(* Logix 5000 AddOnInstructionDefinition export AMCI_3601_AOP_Absolute_Move; software revision 20.03 *)

ADD_ON_INSTRUCTION AMCI_3601_AOP_Absolute_Move   (* revision 0.0, vendor AMCI, ExecuteEnableInFalse *)
// Revision note:
// 3/2020: Version 0 is the initial release
VAR_INPUT
   Axis_Status_Bits : INT; {required}
   _0_normal_1_S_Curve_Acceleration : BOOL;
   _0_Triangular_1_Trapezoidal_S_Curve : BOOL;
   _0_Target_Move_1_Encoder_Move : BOOL;
   Target_Position : DINT; {required}
   Programmed_Speed : DINT; {required}
   Acceleration : INT; {required}
   Deceleration : INT; {required}
END_VAR
VAR_OUTPUT
   EN : BOOL; {access Read Only, visible}
   ER : BOOL; {access Read Only, visible}
END_VAR
VAR_IN_OUT
   AMCI_3601_output_data : AM:1769_3601:O:0; {required}
END_VAR
VAR
   Upper_Result_X_1000 : DINT;
   command_data_block : INT[10];
        [0]   // Command Bits MSW
        [1]   // Command Bits LSW
        [2]   // Upper Target Position
        [3]   // Lower Target Position
        [4]   // Upper Programmed Speed
        [5]   // Lower Programmed Speed
END_VAR

ROUTINE EnableInFalse   (* ladder *)
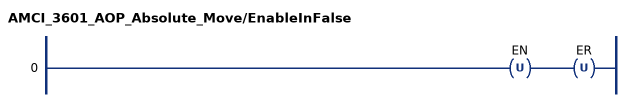
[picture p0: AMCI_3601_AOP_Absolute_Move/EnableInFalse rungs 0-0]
   0: OTU(EN)OTU(ER);
END_ROUTINE

ROUTINE Logic   (* ladder *)
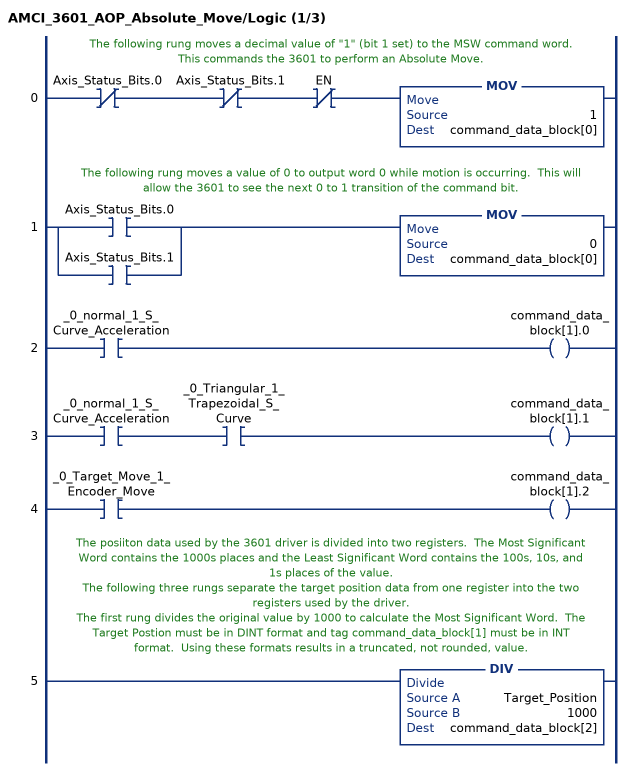
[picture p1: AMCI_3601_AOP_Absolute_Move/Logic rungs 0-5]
   // The following rung moves a decimal value of "1" (bit 1 set) to the MSW command word.  This commands the 3601 to perform an Absolute Move.
   0: XIO(Axis_Status_Bits.0)XIO(Axis_Status_Bits.1)XIO(EN)MOV(1,command_data_block[0]);
   // The following rung moves a value of 0 to output word 0 while motion is occurring.  This will allow the 3601 to see the next 0 to 1 transition of the command bit.
   1: [XIC(Axis_Status_Bits.0) ,XIC(Axis_Status_Bits.1) ]MOV(0,command_data_block[0]);
   2: XIC(_0_normal_1_S_Curve_Acceleration)OTE(command_data_block[1].0);
   3: XIC(_0_normal_1_S_Curve_Acceleration)XIC(_0_Triangular_1_Trapezoidal_S_Curve)OTE(command_data_block[1].1);
   4: XIC(_0_Target_Move_1_Encoder_Move)OTE(command_data_block[1].2);
   // The posiiton data used by the 3601 driver is divided into two registers.  The Most Significant Word contains the 1000s places and the Least Significant Word contains the 100s, 10s, and 1s places of the value.
   // The following three rungs separate the target position data from one register into the two registers used by the driver.
   // The first rung divides the original value by 1000 to calculate the Most Significant Word.  The Target Postion must be in DINT format and tag command_data_block[1] must be in INT format.  Using these formats results in a truncated, not rounded, value.
   5: DIV(Target_Position,1000,command_data_block[2]);
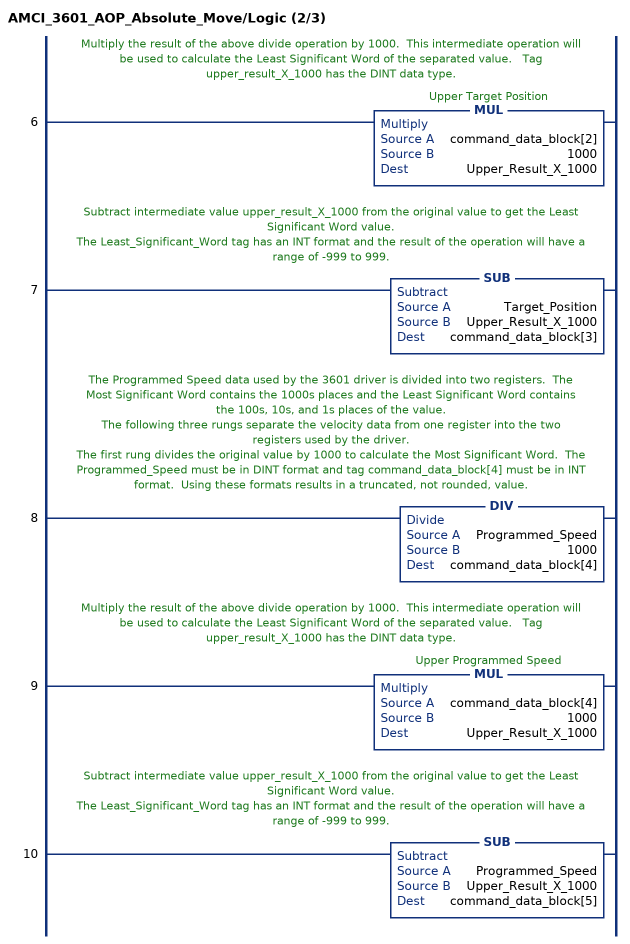
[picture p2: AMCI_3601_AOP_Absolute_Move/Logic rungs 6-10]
   // Multiply the result of the above divide operation by 1000.  This intermediate operation will be used to calculate the Least Significant Word of the separated value.   Tag upper_result_X_1000 has the DINT data type.
   6: MUL(command_data_block[2],1000,Upper_Result_X_1000);
   // Subtract intermediate value upper_result_X_1000 from the original value to get the Least Significant Word value.
   // The Least_Significant_Word tag has an INT format and the result of the operation will have a range of -999 to 999.
   7: SUB(Target_Position,Upper_Result_X_1000,command_data_block[3]);
   // The Programmed Speed data used by the 3601 driver is divided into two registers.  The Most Significant Word contains the 1000s places and the Least Significant Word contains the 100s, 10s, and 1s places of the value.
   // The following three rungs separate the velocity data from one register into the two registers used by the driver.
   // The first rung divides the original value by 1000 to calculate the Most Significant Word.  The Programmed_Speed must be in DINT format and tag command_data_block[4] must be in INT format.  Using these formats results in a truncated, not rounded, value.
   8: DIV(Programmed_Speed,1000,command_data_block[4]);
   // Multiply the result of the above divide operation by 1000.  This intermediate operation will be used to calculate the Least Significant Word of the separated value.   Tag upper_result_X_1000 has the DINT data type.
   9: MUL(command_data_block[4],1000,Upper_Result_X_1000);
   // Subtract intermediate value upper_result_X_1000 from the original value to get the Least Significant Word value.
   // The Least_Significant_Word tag has an INT format and the result of the operation will have a range of -999 to 999.
   10: SUB(Programmed_Speed,Upper_Result_X_1000,command_data_block[5]);
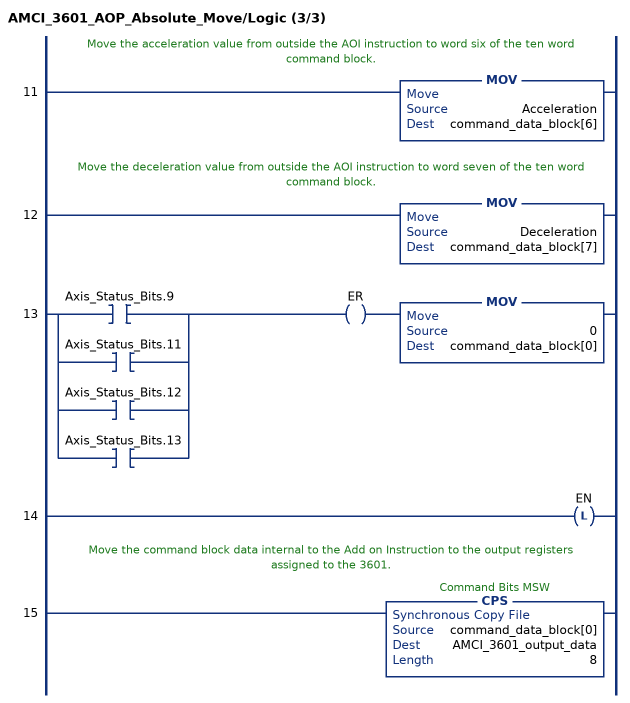
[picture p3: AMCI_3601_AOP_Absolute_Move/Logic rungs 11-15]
   // Move the acceleration value from outside the AOI instruction to word six of the ten word command block.
   11: MOV(Acceleration,command_data_block[6]);
   // Move the deceleration value from outside the AOI instruction to word seven of the ten word command block.
   12: MOV(Deceleration,command_data_block[7]);
   13: [XIC(Axis_Status_Bits.9) ,XIC(Axis_Status_Bits.11) ,XIC(Axis_Status_Bits.12) ,XIC(Axis_Status_Bits.13) ]OTE(ER)MOV(0,command_data_block[0]);
   14: OTL(EN);
   // Move the command block data internal to the Add on Instruction to the output registers assigned to the 3601.
   15: CPS(command_data_block[0],AMCI_3601_output_data,8);
END_ROUTINE
END_ADD_ON_INSTRUCTION
